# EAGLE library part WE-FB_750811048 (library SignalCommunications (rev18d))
WE-FB Flyback Transformer suitable for LT3573/ LT3574/ LT3575/ LT3748 Characteristics easy design in solution less external components needed small board space low cost no optocoupler needed! long term reliability voltage control no aging same external parts for different output voltages easy design of custom power supply due to standard circuit and change of transformers and two components for feedback loop Isolation voltage up to 2.5 kV Applications Isolated power design Sensor interfaces Isolated telecom converters Power over Ethernet Details see: http://katalog.we-online.de/en/pbs/WE-FB_Linear? Updated 2015-04-03 2015 (C) Wurth Elektronik
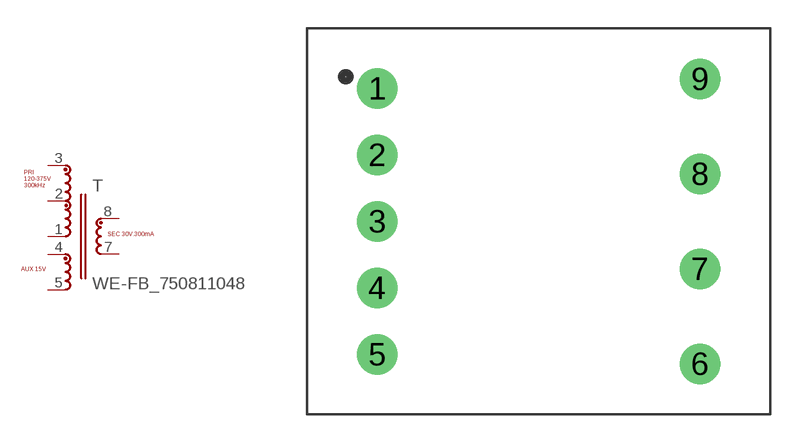
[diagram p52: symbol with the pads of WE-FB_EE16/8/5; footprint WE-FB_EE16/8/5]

Designator prefix T

## WE-FB_750811048_750811048  [WE-FB_EE16/8/5]
1  6  pas
2  7  pas
3  1  pas
4  5  pas
5  4  pas
7  3  pas
8  2  pas

## Footprint WE-FB_EE16/8/5 (pad centres in mm)
drill 1.42: 1 -8.5,7; 2 -8.5,3.5; 3 -8.5,0; 4 -8.5,-3.5; 5 -8.5,-7; 6 8.5,-7.5; 7 8.5,-2.5; 8 8.5,2.5; 9 8.5,7.5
